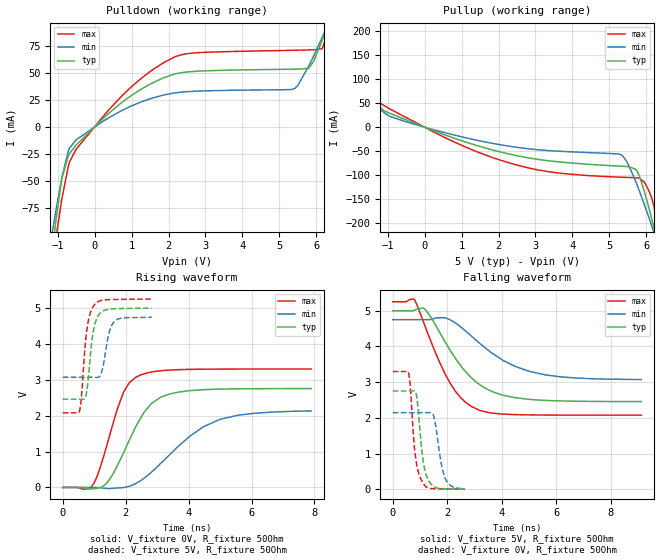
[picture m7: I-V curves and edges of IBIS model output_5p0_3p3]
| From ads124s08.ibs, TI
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|   output_5p0_3p3 Model
[Model]   output_5p0_3p3
Model_type   Output
Polarity   Non-Inverting
Vmeas = 2.5
Vref = 0
Cref = 2pF
Rref = 70
|   typ   min   max
|   (nom PVT)   (fast PVT)   (slow PVT)
C_comp   3.234e-12   3.122e-12   3.353e-12
| Where nom  PVT is Nominal Process, 5V, 27C
|   Fast PVT is Strong Process,  5.25V, -50C
|   Slow PVT is Weak Process,   4.75V, 125C
[Voltage Range]   5   4.75   5.25
|Junction Temperature
[Temperature Range]   27   125   -50
[Pullup Reference]   5   4.75   5.25
[Pulldown Reference]   0   0   0
[Power Clamp Reference]   5   4.75   5.25
[GND Clamp Reference]   0   0   0
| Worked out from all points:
|   slope of the pulldown table from 0 to 0.75 V, typ, clamps not added: 32.7 ohm
|   slope of the pullup table from 0 to 0.75 V, typ, clamps not added: 34.9 ohm
|   falling waveform, V_fixture 5V, R_fixture 50Ohm: 20-80 % time 1.48ns typ, 1.92ns min, 1.17ns max; typ from 5 V to 2.46 V
|   rising waveform, V_fixture 0V, R_fixture 50Ohm: 20-80 % time 987ps typ, 1.69ns min, 698ps max; typ from 0 V to 2.75 V
|   rising waveform, V_fixture 5V, R_fixture 50Ohm: 20-80 % time 199ps typ, 216ps min, 197ps max; typ from 2.46 V to 4.99 V
|   falling waveform, V_fixture 0V, R_fixture 50Ohm: 20-80 % time 237ps typ, 279ps min, 220ps max; typ from 2.75 V to 0.01 V
[Pulldown]
|   Voltage   I(typ)   I(min)   I(max)
-5V       -1.425A    -1.08A     -1.771A
-1.16V    -119.2mA   -100.1mA   -147mA
-1.015V   -78.19mA   -70.86mA   -95.57mA
-720mV    -27.41mA   -23.12mA   -37.56mA
-497mV    -16.44mA   -11.66mA   -20.31mA
905mV     27.09mA    18.18mA    34.43mA
2.225V    49.61mA    31.92mA    65.71mA
5.412V    53.62mA    35.7mA     71.12mA
5.79V     54.4mA     56.23mA    71.41mA
6.162V    80.92mA    83.39mA    72.89mA
6.403V    104.4mA    102.3mA    95.38mA
10V       508.4mA    415.8mA    608.3mA
[Pullup]
|   Voltage   I(typ)   I(min)   I(max)
-5V       423.9mA    339.6mA    534.5mA
-2.473V   163.8mA    135.3mA    202.2mA
-1.335V   51.05mA    46.44mA    59.22mA
-497mV    15.05mA    10.92mA    19.97mA
1.09V     -30.47mA   -21.72mA   -40.73mA
2.481V    -59.12mA   -41.74mA   -78.43mA
5.322V    -81.19mA   -57.63mA   -104mA
5.76V     -93.15mA   -122.3mA   -105.4mA
5.945V    -133.2mA   -160.7mA   -114.5mA
6.204V    -208.4mA   -218.2mA   -163.7mA
6.33V     -247.9mA   -247.6mA   -209.5mA
10V       -1.505A    -1.205A    -1.757A
[Ramp]
R_load = 50
|   typ   min   max
dV/dt_r   1.65274/9.88217e-10   1.28859/1.71858e-09   1.97902/6.97705e-10
dV/dt_f   1.52589/1.47794e-09   1.00955/1.93733e-09   1.90333/1.17475e-09
[Falling Waveform]
V_fixture = 5V
V_fixture_min = 4.75V
V_fixture_max = 5.25V
R_fixture = 50Ohm
|   Time   V(typ)   V(min)   V(max)
0s        5V         4.75V      5.25V
799.3ps   5.014V     4.75V      5.305V
1.211ns   5.017V     4.75V      4.52V
1.929ns   4.122V     4.801V     3.225V
2.475ns   3.486V     4.561V     2.584V
2.891ns   3.124V     4.289V     2.319V
3.669ns   2.732V     3.801V     2.135V
5.01ns    2.521V     3.306V     2.086V
6.695ns   2.469V     3.119V     2.079V
9.128ns   2.458V     3.073V     2.078V
[Rising Waveform]
V_fixture = 0V
V_fixture_min = 0V
V_fixture_max = 0V
R_fixture = 50Ohm
|   Time   V(typ)   V(min)   V(max)
0s        2.363nV    3.266nV    2.146nV
959.9ps   -38.85mV   144.2uV    74.92mV
1.408ns   134mV      -30.31mV   1.193V
1.929ns   958.4mV    -2.136mV   2.644V
2.106ns   1.296V     29.78mV    2.905V
2.475ns   1.928V     189.3mV    3.132V
3.123ns   2.516V     676mV      3.248V
4.042ns   2.695V     1.429V     3.288V
5.01ns    2.738V     1.899V     3.295V
7.901ns   2.753V     2.13V      3.298V
[Rising Waveform]
V_fixture = 5V
V_fixture_min = 4.75V
V_fixture_max = 5.25V
R_fixture = 50Ohm
|   Time   V(typ)   V(min)   V(max)
0s        2.457V     3.067V     2.078V
538.4ps   2.457V     3.067V     2.141V
595.4ps   2.456V     3.067V     2.527V
770.1ps   2.71V      3.068V     4.406V
914.8ps   3.989V     3.067V     4.947V
1.012ns   4.512V     3.066V     5.09V
1.225ns   4.883V     3.173V     5.208V
1.453ns   4.957V     4.239V     5.229V
1.63ns    4.974V     4.609V     5.233V
2.83ns    4.991V     4.738V     5.245V
[Falling Waveform]
V_fixture = 0V
V_fixture_min = 0V
V_fixture_max = 0V
R_fixture = 50Ohm
|   Time   V(typ)   V(min)   V(max)
0s        2.755V     2.148V     3.298V
582.3ps   2.755V     2.148V     3.258V
649.4ps   2.754V     2.148V     2.844V
770.1ps   2.758V     2.148V     1.412V
874.4ps   2.625V     2.148V     721.9mV
1.122ns   773.3mV    2.148V     165.5mV
1.509ns   84.89mV    2.045V     21.25mV
1.772ns   24.47mV    768.3mV    15.82mV
1.985ns   16.16mV    223.3mV    13.26mV
2.649ns   9.72mV     17.27mV    7.88mV
